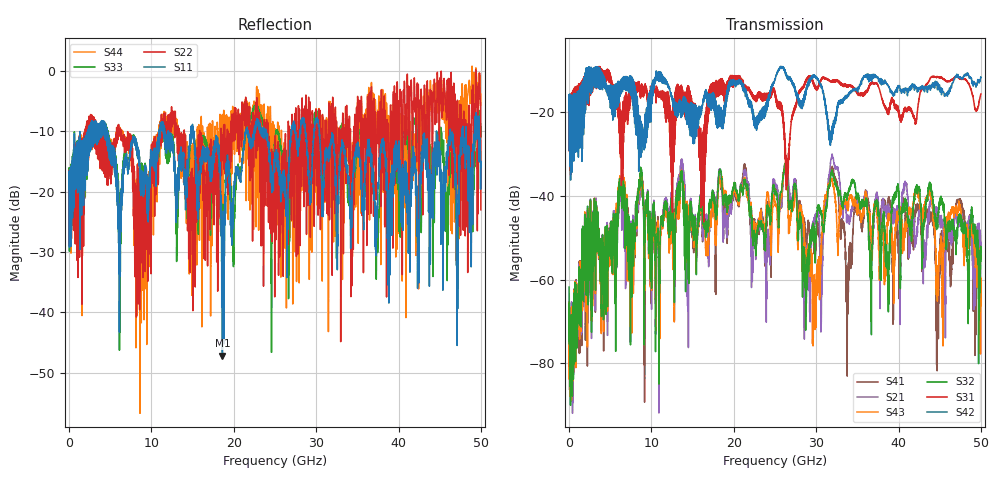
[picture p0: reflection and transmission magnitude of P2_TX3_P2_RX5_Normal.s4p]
!Keysight Technologies,N5225B,MY57041031,A.13.20.10
!Date: Friday, May 31, 2019 11:34:19
!Correction: S11(Full 4 Port(1,2,3,4))
!S12(Full 4 Port(1,2,3,4))
!S13(Full 4 Port(1,2,3,4))
!S14(Full 4 Port(1,2,3,4))
!S21(Full 4 Port(1,2,3,4))
!S22(Full 4 Port(1,2,3,4))
!S23(Full 4 Port(1,2,3,4))
!S24(Full 4 Port(1,2,3,4))
!S31(Full 4 Port(1,2,3,4))
!S32(Full 4 Port(1,2,3,4))
!S33(Full 4 Port(1,2,3,4))
!S34(Full 4 Port(1,2,3,4))
!S41(Full 4 Port(1,2,3,4))
!S42(Full 4 Port(1,2,3,4))
!S43(Full 4 Port(1,2,3,4))
!S44(Full 4 Port(1,2,3,4))
!S4P File: Measurements: <S11,S12,S13,S14>,
!<S21,S22,S23,S24>,
!<S31,S32,S33,S34>,
!<S41,S42,S43,S44>:
# Hz S  dB  R 50.0
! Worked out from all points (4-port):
!   5000 points, 10 MHz to 50 GHz, reference 50 ohm
!   strongest paths, dB at 10 MHz, 12.51 GHz, 25.01 GHz, 37.51 GHz, 50 GHz:
!     S42: -19.5, -16.9, -12.0, -11.6, -11.6
!     S31: -19.6, -42.7, -16.0, -13.6, -15.6
!     S32: -61.8, -41.7, -39.3, -43.1, -55.6
!     S43: -68.7, -43.5, -41.7, -46.7, -63.0
!     S21: -65.2, -40.7, -37.5, -40.9, -54.0
!     S41: -67.0, -42.4, -37.9, -41.1, -53.3
!   lowest |S11| = -47.2 dB at 18.62 GHz (marker M1), VSWR 1.01, Z = 49.7 - j0.345 ohm
!   |S11| at or under -10 dB: 4.63 GHz to 10.95 GHz (6.318 GHz wide, 81.1 % of centre); 15.14 GHz to 21.46 GHz (6.326 GHz wide, 34.6 % of centre); 30.38 GHz to 44.61 GHz (14.23 GHz wide, 37.9 % of centre)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
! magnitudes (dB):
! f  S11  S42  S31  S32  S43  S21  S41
! 10 MHz  -19.6  -19.5  -19.6  -61.8  -68.7  -65.2  -67.0
! 6.36 GHz  -21.8  -12.1  -37.5  -39.5  -36.8  -42.6  -38.7
! 18.62 GHz  -47.2  -22.2  -12.3  -39.6  -37.2  -43.3  -38.9
! 29.78 GHz  -9.6  -11.4  -13.3  -51.2  -58.8  -47.5  -52.7
! 31.82 GHz  -11.2  -25.5  -12.5  -34.8  -35.8  -31.2  -33.7
! 33.8 GHz  -16.4  -16.0  -13.6  -39.9  -42.2  -44.9  -66.8
! 50 GHz  -15.9  -11.6  -15.6  -55.6  -63.0  -54.0  -53.3
